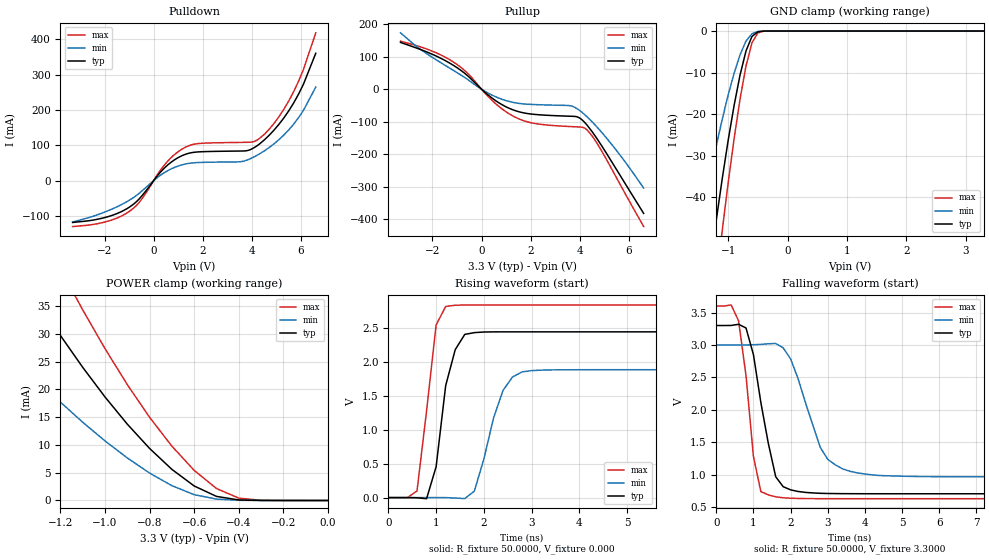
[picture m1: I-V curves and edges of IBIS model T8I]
| IBIS file t8i.ibs created by s2ibis2 version 1.1
| North Carolina State University Electronics Research Laboratory  1995
[IBIS ver]   2.1
[File name]   t8i.ibs
[File Rev]   1.0
[Date]   Wednesday, March 29, 2000
[Source]   From silicon level SPICE at TOSHIBA.
[Notes]   This model does not include the values of Package Model
[Disclaimer]   None.
[Copyright]   Copyright(C) TOSHIBA Corp. 1996-2000. All Rights Reserved
|   Component TC260C
[Component]   TC260C
[Manufacturer]   TOSHIBA
[Package]
| variable   typ   min   max
R_pkg   1.0000f   NA   NA
L_pkg   1.0000fH   NA   NA
C_pkg   1.0000fF   NA   NA
[Pin]  signal_name   model_name   R_pin   L_pin   C_pin
Z   Z   T8I
VDDS   VDDS   POWER
VSS   VSS   GND
| Models and submodels in the file (1): T8I (3-state)
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|   Model T8I
[Model]   T8I
Model_type   3-state
Polarity   Non-Inverting
C_comp   4.2000pF   NA   NA
Vmeas = 1.40V
|Variable   typ   min   max
[Voltage range]  3.3   3.0   3.6
[Temperature Range]   25.0000   100.0000   0.000
[Pullup Reference]   3.3000V   3.0000V   3.6000V
[Pulldown Reference]   0.000V   0.000V   0.000V
[POWER Clamp Reference]   3.3000V   3.0000V   3.6000V
[GND Clamp Reference]   0.000V   0.000V   0.000V
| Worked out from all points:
|   slope of the pulldown table from 0 to 0.495 V, typ, clamps not added: 12.6 ohm
|   slope of the pullup table from 0 to 0.495 V, typ, clamps not added: 15.9 ohm
|   GND clamp passes 1 mA (typ) near -0.57 V on its own axis
|   POWER clamp passes 1 mA (typ) near -0.51 V on its own axis
|   rising waveform, R_fixture 50.0000, V_fixture 0.000: 20-80 % time 309ps typ, 446ps min, 277ps max; typ from 0 V to 2.44 V
|   falling waveform, R_fixture 50.0000, V_fixture 3.3000: 20-80 % time 482ps typ, 723ps min, 334ps max; typ from 3.3 V to 0.707 V
[Pulldown]
| voltage   I(typ)   I(min)   I(max)
-3.3V     -118.3mA   -116.9mA   -130mA
-1.9V     -102.8mA   -86.4mA    -115.5mA
-1V       -75.54mA   -55.79mA   -87.46mA
-500mV    -44.75mA   -30.6mA    -53.64mA
500mV     39.75mA    25.37mA    49.36mA
1.3V      74.6mA     47.15mA    94.71mA
3.6V      83.8mA     54.14mA    108.2mA
4.3V      103.2mA    75.18mA    118.9mA
4.9V      142.9mA    104.1mA    161.7mA
5.5V      197.4mA    143.4mA    225.3mA
6.1V      272.9mA    199mA      314.5mA
6.6V      360.2mA    264.6mA    418.1mA
[Pullup]
| voltage   I(typ)   I(min)   I(max)
-3.3V     143.7mA    173.2mA    147.6mA
-2.1V     110.3mA    102.6mA    119.7mA
-1.1V     71.13mA    55.65mA    81.26mA
-500mV    36.79mA    26.25mA    43.92mA
500mV     -31.32mA   -20.74mA   -39.42mA
1.4V      -66.49mA   -42.11mA   -86.94mA
2.2V      -77.59mA   -47.25mA   -105.6mA
3.6V      -82.91mA   -50.53mA   -114.6mA
3.9V      -84.89mA   -60.4mA    -115.6mA
4.2V      -102.1mA   -78.17mA   -119.4mA
4.9V      -174.8mA   -133.2mA   -191mA
6.6V      -381.4mA   -303.5mA   -421.8mA
[GND_clamp]
| voltage   I(typ)   I(min)   I(max)
-3.3V     -292.8mA   -217.8mA   -337.5mA
-1.5V     -77.97mA   -49.07mA   -98.95mA
-1.3V     -55.88mA   -34.36mA   -72.74mA
-1.2V     -45.43mA   -27.57mA   -60.12mA
-1.1V     -35.51mA   -21.22mA   -47.98mA
-900mV    -17.87mA   -10.14mA   -25.85mA
-800mV    -10.56mA   -5.698mA   -16.34mA
-700mV    -4.792mA   -2.412mA   -8.394mA
-600mV    -1.302mA   -649uA     -2.833mA
-500mV    -170.7uA   -108.2uA   -443.3uA
-400mV    -13.58uA   -13.64uA   -33.16uA
3.3V      153.9pA    4.45uA     -1.048nA
[POWER_clamp]
| voltage   I(typ)   I(min)   I(max)
-3.3V     189.1mA    135.9mA    229.2mA
-1.7V     62.57mA    39.06mA    82.98mA
-1.6V     55.54mA    34.4mA     74.31mA
-1.3V     35.75mA    21.56mA    49.45mA
-1.2V     29.69mA    17.7mA     41.7mA
-1.1V     23.96mA    14.08mA    34.3mA
-900mV    13.74mA    7.658mA    20.85mA
-800mV    9.367mA    4.936mA    14.97mA
-600mV    2.612mA    1.048mA    5.42mA
-500mV    737.5uA    251.8uA    2.156mA
-400mV    94.87uA    37.87uA    425.3uA
0V        153.9pA    711.8pA    166.4pA
[Ramp]
| variable   typ   min   max
dV/dt_r   1.4621/0.2443n   1.1280/0.4084n   1.6995/0.1826n
dV/dt_f   1.5557/0.3972n   1.2187/0.7527n   1.7813/0.2779n
R_load = 50.0000
[Rising Waveform]
R_fixture = 50.0000
V_fixture = 0.000
V_fixture_min = 0.000
V_fixture_max = 0.000
| time   V(typ)   V(min)   V(max)
0s        0V         0V         0V
600ps     -2.802mV   21.22uV    98.23mV
800ps     -16.31mV   134.8uV    1.276V
1ns       454mV      339uV      2.538V
1.2ns     1.647V     -355.1uV   2.81V
1.4ns     2.175V     -6.535mV   2.828V
1.8ns     2.425V     95.05mV    2.833V
2.4ns     2.437V     1.576V     2.833V
2.8ns     2.437V     1.848V     2.833V
10ns      2.437V     1.88V      2.833V
[Falling Waveform]
R_fixture = 50.0000
V_fixture = 3.3000
V_fixture_min = 3.0000
V_fixture_max = 3.6000
| time   V(typ)   V(min)   V(max)
0s        3.3V       3V         3.6V
600ps     3.319V     3V         3.373V
800ps     3.262V     3.001V     2.529V
1ns       2.852V     3.004V     1.283V
1.2ns     2.113V     3.01V      740.8mV
1.6ns     969.3mV    3.023V     660mV
1.8ns     816.4mV    2.956V     645.4mV
2.8ns     714.2mV    1.421V     631.6mV
3.4ns     709mV      1.091V     631.2mV
10ns      707.2mV    968.7mV    631.2mV
